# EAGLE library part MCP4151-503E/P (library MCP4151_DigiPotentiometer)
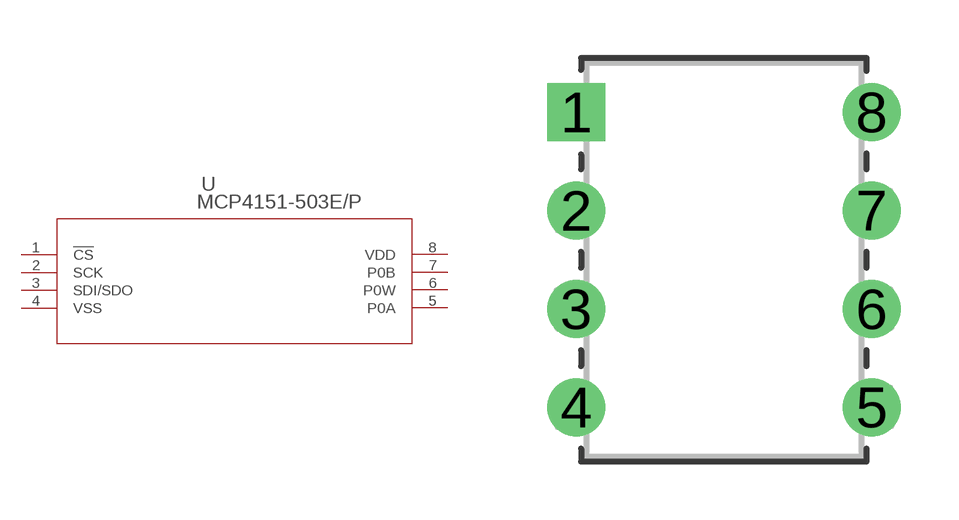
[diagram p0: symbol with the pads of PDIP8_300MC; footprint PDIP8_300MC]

Designator prefix U

## MCP4151-503E/PMCP4151 (MANUFACTURER_PART_NUMBER: MCP4151503EP; VENDOR: Microchip)  [PDIP8_300MC]
1  !CS  pas
2  SCK  pas
3  SDI/SDO  pas
4  VSS  pas
5  P0A  pas
6  P0W  pas
7  P0B  pas
8  VDD  pas

## Footprint PDIP8_300MC (pad centres in mm)
drill 0.991 pad 1.499 square: 1 -7.62,7.62
drill 0.991 pad 1.499: 2 -7.62,5.08; 3 -7.62,2.54; 4 -7.62,0; 5 0,0; 6 0,2.54; 7 0,5.08; 8 0,7.62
